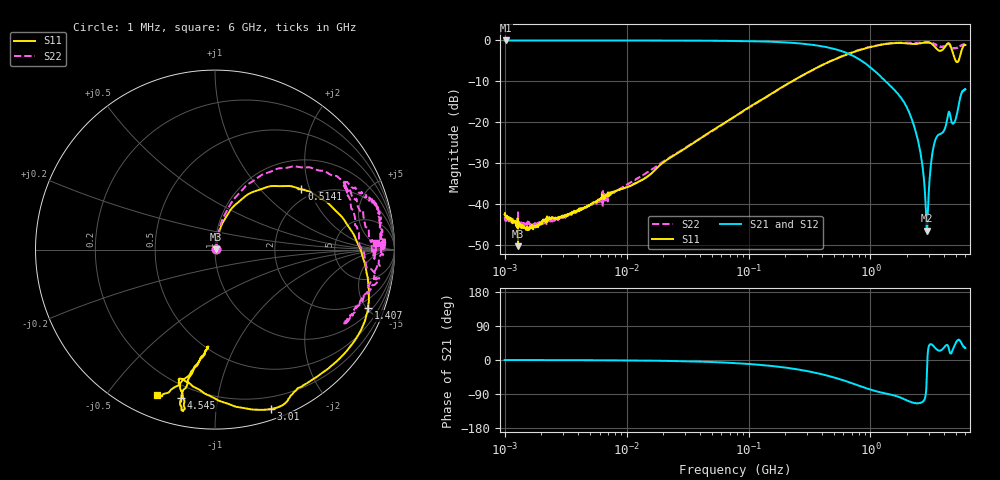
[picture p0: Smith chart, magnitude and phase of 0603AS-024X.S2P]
!s-Parameter Generated by FASTRON Sdn. Bhd.
!FASTRON P/N : 0603AS-024X
!Keysight Technologies: E5071C_MY46733604_B.14.02
!Date: Thu Nov 23 10:40:49 2023
!Version  :Rev01  Thu Nov 23 10:40:49 2023
!Data & Calibration Information:
!Freq  S11:SOLT2(ON)  S21:SOLT2(ON)  S12:SOLT2(ON)  S22:SOLT2(ON)
!PortZ  Port1:50+j0  Port2:50+j0
!When reading reference impedance value at option line is always used.
! Remarks : This data is being provided solely for informational purposes.
# Hz S dB R 50
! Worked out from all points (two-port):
!   1601 points, 1 MHz to 6 GHz, reference 50 ohm
!   highest |S21| = -0.04 dB at 1.032 MHz (marker M1); lowest = -46.5 dB at 2.907 GHz (marker M2)
!   |S21| within 3 dB of the highest: start of sweep to 631 MHz
!   lowest |S11| = -50.3 dB at 1.288 MHz (marker M3), VSWR 1.01, Z = 50.3 + j0.117 ohm
!   |S11| at or under -10 dB: start of sweep to 228.1 MHz
!   |S22| runs from -45.9 to -0.4 dB; largest |S21 - S12| = 0.0073
!   S11 on the Smith chart (normalised r, x): 1 MHz: 1.01, +0.01; 514.1 MHz: 1.72, +1.76; 1.407 GHz: 1.31, -5.10; 3.01 GHz: 0.09, -1.41; 4.545 GHz: 0.13, -0.79; 6 GHz: 0.10, -0.67
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1000000  -42.52 21.2  -0.05 -0.1  -0.05 -0.1  -43.19 21.2
1031961  -43.32 14.6  -0.04 -0.1  -0.05 -0.1  -43.43 13.7
1287650  -50.31 22.4  -0.06 -0.1  -0.04 -0.0  -42.04 12.3
4277066  -41.38 56.9  -0.05 -0.5  -0.05 -0.5  -41.28 57.4
1.823719e7  -30.88 76.8  -0.06 -2.0  -0.07 -2.0  -30.42 75.0
7.757876e7  -18.56 76.3  -0.15 -8.1  -0.16 -8.1  -18.62 78.0
3.307917e8  -7.34 52.1  -1.08 -31.8  -1.08 -31.8  -7.41 61.8
5.140627e8  -4.62 34.9  -2.17 -47.0  -2.16 -47.0  -4.63 50.7
8.707108e8  -2.12 4.9  -5.28 -71.6  -5.28 -71.6  -2.02 31.2
1.407106e9  -0.79 -20.9  -10.72 -90.3  -10.73 -90.3  -0.80 16.8
1.414819e9  -0.78 -21.1  -10.80 -90.5  -10.82 -90.5  -0.78 16.7
2.226311e9  -0.89 -56.0  -20.08 -112.2  -20.07 -112.1  -0.60 5.1
2.584893e9  -0.70 -63.1  -27.95 -113.0  -27.93 -112.8  -0.57 0.4
2.907198e9  -0.48 -67.6  -46.49 -24.3  -46.50 -24.0  -0.46 3.4
3.00975e9  -0.53 -70.7  -36.72 36.7  -36.69 36.7  -0.50 3.0
3.141603e9  -0.75 -76.5  -29.94 41.4  -29.91 41.3  -0.67 -1.2
3.280226e9  -1.22 -84.3  -26.24 37.3  -26.22 37.2  -0.70 -5.3
3.806705e9  -2.51 -105.7  -22.74 25.9  -22.74 25.8  -1.65 -28.9
4.292686e9  -0.82 -101.1  -18.72 38.5  -18.75 38.5  -0.92 -12.8
4.545048e9  -1.42 -102.8  -18.92 17.5  -18.94 17.5  -1.64 -0.3
5.048685e9  -5.21 -94.0  -18.65 47.9  -18.66 48.0  -1.85 27.8
6e9  -1.16 -111.7  -11.98 31.6  -11.98 31.7  -0.93 2.4
